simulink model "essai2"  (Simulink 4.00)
settings: Solver=ode45  SolverMode=SingleTasking  StartTime=0.0  StopTime=50*delt  FixedStep=[]  MaxStep=1  RelTol=1e-3  AbsTol=1e-3
PreLoadFcn:
  | demo2dat
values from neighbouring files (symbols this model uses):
  delt = 0.2    [demo1dat.m]    (also in essai1dat.m; essai2dat.m = 0.1)
  m = 4    [demo1dat.m]    (also in demo2dat.m = 3; essai1dat.m; essai2dat.m = 6; mynlcmpc.m = mp(1:max(size(mp))-1))
  model = tfd2step(1.6,delt,1,g)    [essai2dat.m]    (also in mynlcmpc.m = modelpd(:,1:nu); mynlcmpc2.m = modelpd(:,1:nu); mynlcmpc3.m = modelpd(:,1:nu); scrtp1.m = tfd2step(tfinal,Ts,1,g))
  p = 10    [demo1dat.m]    (also in demo2dat.m; essai1dat.m; essai2dat.m; mynlcmpc.m = mp(max(size(mp))))
  r = [68.3 2]    [demo1dat.m]    (also in demo2dat.m = [0 0 0]; essai1dat.m; essai2dat.m = 10; mynlcmpc.m = zeros(1,ny))
  uwt = [0 0]    [demo1dat.m]    (also in demo2dat.m = 0.6*[1 1]; essai1dat.m; essai2dat.m = 1; mynlcmpc.m = ryuwt(:,2*ny+1:2*ny+nu))
  ywt = [1 1]    [demo1dat.m]    (also in demo2dat.m = [0.2,0,1]; essai1dat.m; essai2dat.m = 1; mynlcmpc.m = ryuwt(:,ny+1:2*ny))

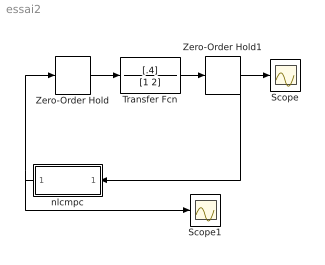
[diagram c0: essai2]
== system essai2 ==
  Scope : Scope
  Scope1 : Scope
  Transfer Fcn : TransferFcn  Numerator=[.4]  Denominator=[1 2]  AbsoluteTolerance=auto  Realization=auto
  Zero-Order Hold : ZeroOrderHold  SampleTime=delt
  Zero-Order Hold1 : ZeroOrderHold  SampleTime=delt
  nlcmpc : Subsystem  Orientation=left  AncestorBlock=nlmpclib/nlcmpc  mask(myCMPC-SIMULINK){modelpd=[model []], ryuwt=[r ywt uwt], mp=[m p], yulim=[[] []], tfilter=[], ud0=[0 []]}
      mask help: Masked MATLAB function block calls nlcmpc, links CMPC and SIMULINK.
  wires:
  Transfer Fcn/1 -> Zero-Order Hold1/1
  nlcmpc/1(Out1) -> Scope1/1, Zero-Order Hold/1
  Zero-Order Hold/1 -> Transfer Fcn/1
  Zero-Order Hold1/1 -> nlcmpc/1(In1), Scope/1

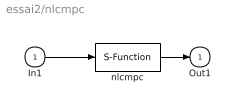
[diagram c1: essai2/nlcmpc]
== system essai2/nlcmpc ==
  In1 : Inport  Port=1  LatchInput=off
  nlcmpc : S-Function  FunctionName=mynlcmpc  Parameters=modelpd,mp,tfilter,ryuwt,ud0,yulim  PortCounts=[]  SFunctionModules=''
  Out1 : Outport  Port=1  InitialOutput=0
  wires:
  In1/1 -> nlcmpc/1
  nlcmpc/1 -> Out1/1
